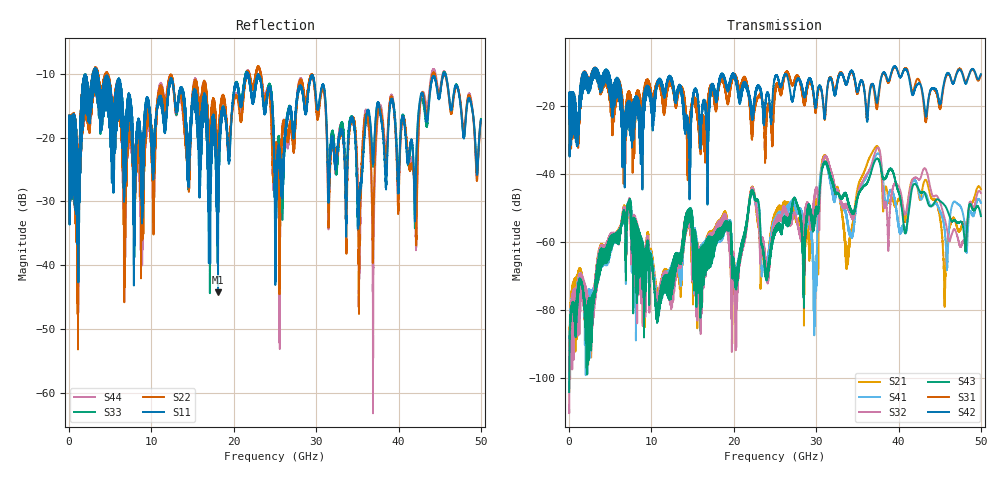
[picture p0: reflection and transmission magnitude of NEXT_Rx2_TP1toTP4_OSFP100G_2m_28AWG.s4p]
! Touchstone data
! Created: 27-Feb-2019 by IdEM 12 (12.1.0)
! COMMENTS
!  Created Wed Feb 27 12:03:36 2019
!  64 Port Network Data from SP1.SP block
!  freq  magS1_1  angS1_1  magS1_2  angS1_2  magS1_3  angS1_3  magS1_4  angS1_4
!  magS1_5  angS1_5  magS1_6  angS1_6  magS1_7  angS1_7  magS1_8  angS1_8
!  magS1_9  angS1_9  magS1_10  angS1_10  magS1_11  angS1_11  magS1_12  angS1_12
!  magS1_13  angS1_13  magS1_14  angS1_14  magS1_15  angS1_15  magS1_16  angS1_16
!  magS1_17  angS1_17  magS1_18  angS1_18  magS1_19  angS1_19  magS1_20  angS1_20
!  magS1_21  angS1_21  magS1_22  angS1_22  magS1_23  angS1_23  magS1_24  angS1_24
!  magS1_25  angS1_25  magS1_26  angS1_26  magS1_27  angS1_27  magS1_28  angS1_28
!  magS1_29  angS1_29  magS1_30  angS1_30  magS1_31  angS1_31  magS1_32  angS1_32
!  magS1_33  angS1_33  magS1_34  angS1_34  magS1_35  angS1_35  magS1_36  angS1_36
!  magS1_37  angS1_37  magS1_38  angS1_38  magS1_39  angS1_39  magS1_40  angS1_40
!  magS1_41  angS1_41  magS1_42  angS1_42  magS1_43  angS1_43  magS1_44  angS1_44
!  magS1_45  angS1_45  magS1_46  angS1_46  magS1_47  angS1_47  magS1_48  angS1_48
!  magS1_49  angS1_49  magS1_50  angS1_50  magS1_51  angS1_51  magS1_52  angS1_52
!  magS1_53  angS1_53  magS1_54  angS1_54  magS1_55  angS1_55  magS1_56  angS1_56
!  magS1_57  angS1_57  magS1_58  angS1_58  magS1_59  angS1_59  magS1_60  angS1_60
!  magS1_61  angS1_61  magS1_62  angS1_62  magS1_63  angS1_63  magS1_64  angS1_64
!  magS2_1  angS2_1  magS2_2  angS2_2  magS2_3  angS2_3  magS2_4  angS2_4
!  magS2_5  angS2_5  magS2_6  angS2_6  magS2_7  angS2_7  magS2_8  angS2_8
!  magS2_9  angS2_9  magS2_10  angS2_10  magS2_11  angS2_11  magS2_12  angS2_12
!  magS2_13  angS2_13  magS2_14  angS2_14  magS2_15  angS2_15  magS2_16  angS2_16
!  magS2_17  angS2_17  magS2_18  angS2_18  magS2_19  angS2_19  magS2_20  angS2_20
!  magS2_21  angS2_21  magS2_22  angS2_22  magS2_23  angS2_23  magS2_24  angS2_24
!  magS2_25  angS2_25  magS2_26  angS2_26  magS2_27  angS2_27  magS2_28  angS2_28
!  magS2_29  angS2_29  magS2_30  angS2_30  magS2_31  angS2_31  magS2_32  angS2_32
!  magS2_33  angS2_33  magS2_34  angS2_34  magS2_35  angS2_35  magS2_36  angS2_36
!  magS2_37  angS2_37  magS2_38  angS2_38  magS2_39  angS2_39  magS2_40  angS2_40
!  magS2_41  angS2_41  magS2_42  angS2_42  magS2_43  angS2_43  magS2_44  angS2_44
!  magS2_45  angS2_45  magS2_46  angS2_46  magS2_47  angS2_47  magS2_48  angS2_48
!  magS2_49  angS2_49  magS2_50  angS2_50  magS2_51  angS2_51  magS2_52  angS2_52
!  magS2_53  angS2_53  magS2_54  angS2_54  magS2_55  angS2_55  magS2_56  angS2_56
!  magS2_57  angS2_57  magS2_58  angS2_58  magS2_59  angS2_59  magS2_60  angS2_60
!  magS2_61  angS2_61  magS2_62  angS2_62  magS2_63  angS2_63  magS2_64  angS2_64
!  magS3_1  angS3_1  magS3_2  angS3_2  magS3_3  angS3_3  magS3_4  angS3_4
!  magS3_5  angS3_5  magS3_6  angS3_6  magS3_7  angS3_7  magS3_8  angS3_8
!  magS3_9  angS3_9  magS3_10  angS3_10  magS3_11  angS3_11  magS3_12  angS3_12
!  magS3_13  angS3_13  magS3_14  angS3_14  magS3_15  angS3_15  magS3_16  angS3_16
!  magS3_17  angS3_17  magS3_18  angS3_18  magS3_19  angS3_19  magS3_20  angS3_20
!  magS3_21  angS3_21  magS3_22  angS3_22  magS3_23  angS3_23  magS3_24  angS3_24
!  magS3_25  angS3_25  magS3_26  angS3_26  magS3_27  angS3_27  magS3_28  angS3_28
!  magS3_29  angS3_29  magS3_30  angS3_30  magS3_31  angS3_31  magS3_32  angS3_32
!  magS3_33  angS3_33  magS3_34  angS3_34  magS3_35  angS3_35  magS3_36  angS3_36
!  magS3_37  angS3_37  magS3_38  angS3_38  magS3_39  angS3_39  magS3_40  angS3_40
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# Hz S MA R 50
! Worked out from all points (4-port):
!   5000 points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, 10 MHz to 50 GHz, reference 50 ohm
!   strongest paths, dB at 10 MHz, 12.51 GHz, 25.01 GHz, 37.51 GHz, 50 GHz:
!     S42: -18.0, -12.5, -11.5, -17.6, -10.7
!     S31: -18.0, -14.0, -15.8, -18.9, -11.0
!     S43: -104.0, -75.3, -57.0, -35.6, -52.4
!     S32: -107.8, -79.1, -55.1, -32.3, -45.6
!     S41: -103.9, -73.7, -54.0, -33.9, -48.5
!     S21: -103.9, -76.0, -52.4, -32.1, -44.5
!   lowest |S11| = -44.3 dB at 18.09 GHz (marker M1), VSWR 1.01, Z = 49.5 + j0.362 ohm
!   |S11| at or under -10 dB: 3.49 GHz to 21.47 GHz (17.98 GHz wide, 144 % of centre); 21.77 GHz to 45.47 GHz (23.7 GHz wide, 70.5 % of centre); 45.66 GHz to end of sweep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
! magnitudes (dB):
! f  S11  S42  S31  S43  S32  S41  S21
! 10 MHz  -17.7  -18.0  -18.0  -104.0  -107.8  -103.9  -103.9
! 18.09 GHz  -44.3  -14.8  -16.7  -56.2  -54.2  -56.5  -53.9
! 31.06 GHz  -13.1  -23.2  -23.6  -36.7  -35.0  -36.6  -34.7
! 33.78 GHz  -24.6  -13.1  -13.2  -46.9  -49.4  -53.4  -62.9
! 37.37 GHz  -15.2  -19.1  -21.0  -35.5  -32.5  -34.1  -31.8
! 45.62 GHz  -9.9  -12.2  -12.8  -49.2  -53.3  -57.1  -76.1
! 50 GHz  -17.2  -10.7  -11.0  -52.4  -45.6  -48.5  -44.5
